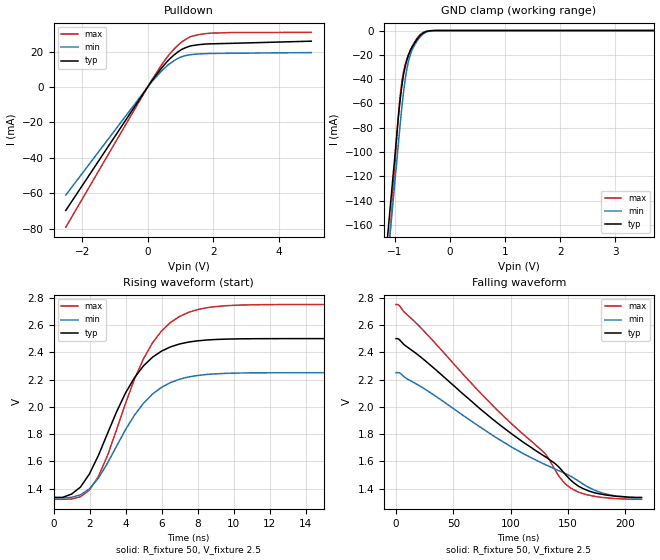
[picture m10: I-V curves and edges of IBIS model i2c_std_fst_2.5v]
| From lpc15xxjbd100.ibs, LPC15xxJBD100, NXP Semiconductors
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[Model]   i2c_std_fst_2.5v
Model_type I/O_open_drain
Vinl=7.500E-01
Vinh=1.750E+00
Vref=2.500E+00
Rref=2.000E+03
Cref=0.000E+00
Vmeas=1.250E+00
C_comp   2.010E-12   2.010E-12   2.010E-12
[Voltage Range]   2.500E+00   2.250E+00   2.750E+00
[POWER Clamp Reference]   2.500E+00   2.250E+00   2.750E+00
[GND Clamp Reference]   0.000E+00   0.000E+00   0.000E+00
[Pullup Reference]   2.500E+00   2.250E+00   2.750E+00
[Pulldown Reference]   0.000E+00   0.000E+00   0.000E+00
[Temperature Range]   25   85   -40
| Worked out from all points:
|   slope of the pulldown table from 0 to 0.375 V, typ, clamps not added: 39.4 ohm
|   GND clamp passes 1 mA (typ) near -0.44 V on its own axis
|   rising waveform, R_fixture 50, V_fixture 2.5: 20-80 % time 2.59ns typ, 2.63ns min, 2.6ns max; typ from 1.34 V to 2.5 V
|   falling waveform, R_fixture 50, V_fixture 2.5: 20-80 % time 105ns typ, 110ns min, 99.6ns max; typ from 2.5 V to 1.34 V
[GND Clamp]
-2.5V     -855.8mA   -864.5mA   -1.076A
-1.02V    -114.5mA   -135.6mA   -125.7mA
-960mV    -84.05mA   -106.2mA   -86.15mA
-920mV    -64.87mA   -86.33mA   -62.54mA
-880mV    -48.71mA   -67.39mA   -45.23mA
-840mV    -36.34mA   -50.69mA   -33.86mA
-780mV    -24.34mA   -31.78mA   -23.51mA
-720mV    -16.88mA   -20.26mA   -16.52mA
-620mV    -8.86mA    -10.44mA   -8.205mA
-480mV    -1.947mA   -2.73mA    -1.503mA
-260mV    0A         0A         0A
5V        0A         0A         0A
[Pulldown]
-2.5V     -69.61mA   -60.98mA   -79.07mA
120mV     3.252mA    2.799mA    3.74mA
400mV     10.13mA    8.598mA    11.78mA
600mV     14.46mA    12.11mA    16.99mA
800mV     17.99mA    14.83mA    21.33mA
1.02V     20.98mA    16.96mA    25.12mA
1.34V     23.3mA     18.34mA    28.62mA
1.78V     24.3mA     18.87mA    30.2mA
2.56V     24.68mA    19.08mA    30.77mA
5V        25.9mA     19.46mA    30.9mA
[Rising Waveform]
R_fixture = 50
V_fixture = 2.5
V_fixture_min = 2.25
V_fixture_max = 2.75
0s        1.336V     1.332V     1.322V
1ns       1.36V      1.337V     1.325V
2ns       1.509V     1.4V       1.391V
3ns       1.805V     1.587V     1.643V
4.5ns     2.214V     1.94V      2.204V
5ns       2.301V     2.027V     2.353V
6ns       2.409V     2.143V     2.556V
7.5ns     2.475V     2.219V     2.692V
11ns      2.499V     2.249V     2.748V
29.5ns    2.5V       2.25V      2.75V
[Falling Waveform]
R_fixture = 50
V_fixture = 2.5
V_fixture_min = 2.25
V_fixture_max = 2.75
0s        2.5V       2.25V      2.75V
21.5ns    2.365V     2.149V     2.581V
87.5ns    1.888V     1.773V     1.982V
129ns     1.64V      1.58V      1.665V
142.5ns   1.554V     1.529V     1.486V
150ns     1.483V     1.501V     1.419V
159.5ns   1.416V     1.454V     1.373V
172ns     1.373V     1.393V     1.345V
190ns     1.346V     1.349V     1.328V
214ns     1.336V     1.332V     1.322V
[Ramp]
dV/dt_r   6.9842E-01/2.5630E-09   5.5101E-01/2.5970E-09   8.5693E-01/2.5820E-09
dV/dt_f   6.9842E-01/1.0545E-07   5.5101E-01/1.0989E-07   8.5693E-01/9.9679E-08
R_load = 50
